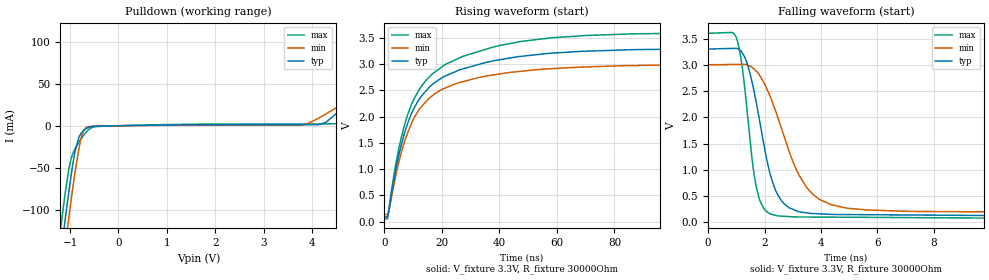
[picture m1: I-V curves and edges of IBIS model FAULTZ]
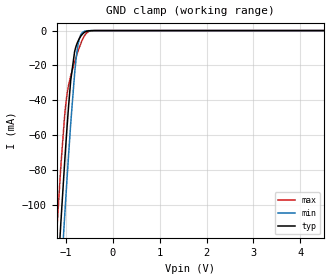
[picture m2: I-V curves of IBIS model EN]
|Texas Instruments Incorporated
| 3.3V to 18V MUX with Overcurrent Limit
| Marketing part#   Digital Voltage Range   Package-type   #pins
| TPS22980RGPR   3.0 - 3.6V   RGP   20
[IBIS Ver]   4.1
[File name]   tps22980.ibs
[File Rev]   1.0
[Date]   12/12/2012
[Source]
| Texas Instruments Incorporated.
| Analog-eLab Design Center, HPA
| 12500 TI Blvd
| Dallas, TX -75243
| e-mail: elab_scm_ibis@list.ti.com
[Notes]   Revision History:
| Rev 1.0: 12/12/2012
| - Initial version of the model
| - Model generated from spice simulations
| - C_comp although listed in numerical order of value are
|   obtained from varying PVT conditions. For PVT conditions for
|   each specific value refer the buffer description under
|   respective [Model]. IBIS model user is responsible for using
|   appropriate C_comp to simulate for Signal Integrity.
[Disclaimer]
| This model is designed as an aid for customers of Texas Instruments.
| TI and its licensors and suppliers make no warranties, either expressed
| or implied, with respect to this  model, including the warranties of
| merchantability or fitness for a particular purpose. The model is
| provided solely on an "as is" basis. The entire risk as to its quality
| and performance is with the customer.
[Copyright]
 (C) Copyright 2012 Texas Instruments Incorporated.All rights reserved.
|   TPS22980
[Component]   TPS22980
[Manufacturer]   TI
[Package]   | 20 pin RGP
| variable   typ   min   max
R_pkg   0.05   0.04   0.06
L_pkg   1nH   0.8nH   1.2nH
C_pkg   0.2pF   0.16pF   0.24pF
[Pin]  signal_name   model_name   R_pin   L_pin   C_pin
1   GND   GND   NA   NA   NA
2   GND   GND   NA   NA   NA
3   GND   GND   NA   NA   NA
4   FAULTZ   FAULTZ   NA   NA   NA
5   EN   EN   NA   NA   NA
6   VHV   NC   NA   NA   NA
7   VHV   NC   NA   NA   NA
8   ISET_V3P3   NC   NA   NA   NA
9   ISET_S3   NC   NA   NA   NA
10   ISET_S0   NC   NA   NA   NA
11   HV_EN   EN   NA   NA   NA
12   OUT   NC   NA   NA   NA
13   GND   GND   NA   NA   NA
14   OUT   NC   NA   NA   NA
15   GND   GND   NA   NA   NA
16   RSVD   NC   NA   NA   NA
17   S0   EN   NA   NA   NA
18   V3P3OUT   NC   NA   NA   NA
19   V3P3   NC   NA   NA   NA
20   V3P3   NC   NA   NA   NA
| Models and submodels in the file (2): FAULTZ (Open_drain), EN (Input)
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|   Model
[Model]   FAULTZ
Model_type   Open_drain
Polarity   Non-Inverting
Vmeas = 1.65
Vref = 3.3
Cref = 1pF
Rref = 30000
|   typ   min   max
C_comp   1.1381pF   1.0022pF   1.2827pF
[Voltage Range]   3.3   3   3.6
[Temperature Range]   27   85   -40
[Pullup Reference]   3.3   3   3.6
[Pulldown Reference]   0   0   0
[Power Clamp Reference]   3.3   3   3.6
[GND Clamp Reference]   0   0   0
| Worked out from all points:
|   slope of the pulldown table from 0 to 0.495 V, typ, clamps not added: 1 kohm
|   falling waveform, V_fixture 3.3V, R_fixture 30000Ohm: 20-80 % time 743ps typ, 1.26ns min, 452ps max; typ from 3.3 V to 0.095 V
|   rising waveform, V_fixture 3.3V, R_fixture 30000Ohm: 20-80 % time 14.7ns typ, 14ns min, 15.7ns max; typ from 0.095 V to 3.3 V
[Pulldown]
|   Voltage   I(typ)   I(min)   I(max)
-3.3V     -1.21A     -1.228A    -1.211A
-1.221V   -167mA     -198.6mA   -134.7mA
-1.102V   -111.9mA   -143.5mA   -80.68mA
-1.033V   -81.4mA    -112.3mA   -54.01mA
-904.2mV  -32.47mA   -57.87mA   -28.17mA
-815.1mV  -13.19mA   -26.26mA   -19.39mA
-706.2mV  -5.002mA   -4.651mA   -10.29mA
-528mV    -830.9uA   -476.7uA   -1.712mA
3.779V    1.285mA    879.6uA    2.127mA
4.293V    4.131mA    14.25mA    2.13mA
4.59V     19mA       24.43mA    2.729mA
6.6V      135.5mA    96.05mA    223.5mA
[Ramp]
R_load = 30000
|   typ   min   max
dV/dt_r   1.92311/1.46749e-08   1.7183/1.40509e-08   2.12226/1.55011e-08
dV/dt_f   1.92311/7.38414e-10   1.7183/1.25483e-09   2.12226/4.49788e-10
[Falling Waveform]
V_fixture = 3.3V
V_fixture_min = 3V
V_fixture_max = 3.6V
R_fixture = 30000Ohm
C_fixture = 0F
|   Time   V(typ)   V(min)   V(max)
0s        3.3V       3V         3.6V
981.9ps   3.314V     3.007V     3.54V
1.298ns   3.148V     3.008V     2.556V
1.623ns   2.514V     2.92V      942.2mV
1.837ns   1.903V     2.791V     415.4mV
2.366ns   646.2mV    2.159V     136.7mV
3.03ns    242.1mV    1.128V     104.4mV
4.366ns   152.5mV    336mV      99.06mV
7.371ns   139.5mV    207.7mV    89.88mV
250ns     94.79mV    136.1mV    62.89mV
[Rising Waveform]
V_fixture = 3.3V
V_fixture_min = 3V
V_fixture_max = 3.6V
R_fixture = 30000Ohm
C_fixture = 0F
|   Time   V(typ)   V(min)   V(max)
0s        94.79mV    136.1mV    62.89mV
1.137ns   96.48mV    132mV      67.33mV
3.904ns   958mV      848.9mV    1.066V
6.573ns   1.593V     1.437V     1.746V
9.132ns   2.012V     1.83V      2.185V
12.09ns   2.325V     2.131V     2.509V
20.89ns   2.763V     2.536V     2.98V
37.38ns   3.054V     2.788V     3.316V
85.22ns   3.271V     2.97V      3.571V
250ns     3.3V       3V         3.6V
|   Model
[Model]   EN
Model_type   Input
Vinl = 0.6
Vinh = 2.7
|   typ   min   max
C_comp   0.90611pF   0.7723pF   1.0265pF
[Voltage Range]   3.3   3   3.6
[Temperature Range]   27   85   -40
[Power Clamp Reference]   3.3   3   3.6
[GND Clamp Reference]   0   0   0
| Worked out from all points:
|   GND clamp passes 1 mA (typ) near -0.60 V on its own axis
[GND Clamp]
|   Voltage   I(typ)   I(min)   I(max)
-3.3V     -1.173A    -1.205A    -1.14A
-1.211V   -156.6mA   -189.6mA   -122mA
-1.112V   -112.1mA   -144.5mA   -79.67mA
-1.102V   -107.8mA   -140mA     -75.71mA
-1.033V   -78.18mA   -109.4mA   -50.78mA
-973.5mV  -54.52mA   -83.97mA   -36.07mA
-894.3mV  -27.96mA   -52.21mA   -25.69mA
-815.1mV  -12.22mA   -25.03mA   -18.09mA
-755.7mV  -6.95mA    -10.56mA   -12.96mA
-617.1mV  -1.271mA   -565.4uA   -3.611mA
-399.3mV  -8.876uA   -4.252uA   -21.47uA
6.6V      0A         0A         0A
[POWER Clamp]
|   Voltage   I(typ)   I(min)   I(max)
-3.3V     0A         0A         0A
-3.28V    0A         0A         0A
-3.27V    0A         0A         0A
6.6V      0A         0A         0A
